PROGRAM MAIN
VAR
	fbProxyTcComIncrementModule	: FB_ProxyTcComIncrementModule(	IID	:= TC_GLOBAL_IID_LIST.IID_IIncrement);
	nValue: INT;
END_VAR

IF fbProxyTcComIncrementModule.ip <> 0 THEN
	
	fbProxyTcComIncrementModule.Cyclic();
	fbProxyTcComIncrementModule.ip.doIncrement(1,ADR(nValue));
	
END_IF

END_PROGRAM
